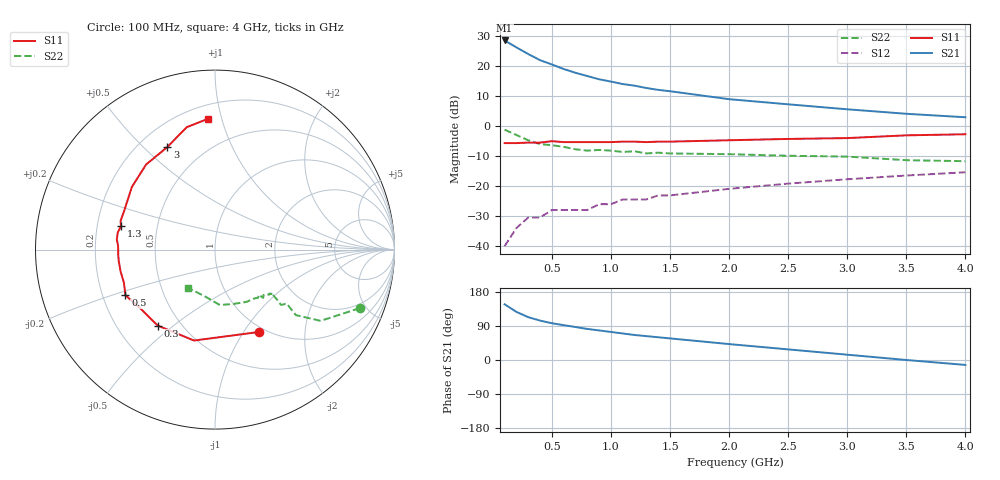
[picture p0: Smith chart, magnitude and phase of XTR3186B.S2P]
! HXTR-3186
! Typical S-Parameters Vce = 10 V, Ic = 15 mA
# ghz s ma r 50
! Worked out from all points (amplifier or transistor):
!   20 points, 100 MHz to 4 GHz, reference 50 ohm
!   highest |S21| = 28.5 dB at 100 MHz (marker M1)
!   |S21| within 3 dB of that: start of sweep to 231.3 MHz
!   unconditionally stable (mu >= 1): 773.1 MHz to 835.6 MHz; 974.3 MHz to 1.031 GHz; 1.205 GHz to 3.226 GHz
!   at 400 MHz: K = 0.67, MSG = 26.2 dB, |S12| = -30.5 dB
!   at 1.1 GHz: K = 0.95, MSG = 19.2 dB, |S12| = -24.4 dB
!   at 4 GHz: K = 0.91, MSG = 9.2 dB, |S12| = -15.4 dB
!   S11 on the Smith chart (normalised r, x): 100 MHz: 0.93, -1.17; 300 MHz: 0.37, -0.44; 500 MHz: 0.30, -0.22; 1.3 GHz: 0.30, +0.11; 3 GHz: 0.31, +0.59; 4 GHz: 0.29, +0.91
0.1  0.52 -62.0  26.6 147.0  0.01 66.0  0.87 -22.0
0.2  0.52 -103.0  20.4 127.0  0.02 55.0  0.71 -34.0
0.3  0.53 -127.0  15.8 113.0  0.03 49.0  0.58 -39.0
0.4  0.53 -142.0  12.5 104.0  0.03 48.0  0.5 -37.0
0.5  0.56 -153.0  10.6 97.0  0.04 47.0  0.48 -40.0
0.6  0.54 -160.0  8.9 92.0  0.04 49.0  0.45 -39.0
0.7  0.54 -167.0  7.7 87.0  0.04 49.0  0.41 -38.0
0.8  0.54 -173.0  6.8 82.0  0.04 50.0  0.39 -39.0
0.9  0.54 -177.0  6 78.0  0.05 51.0  0.4 -38.0
1  0.54 178.0  5.5 74.0  0.05 52.0  0.39 -40.0
1.1  0.55 174.0  5 70.0  0.06 52.0  0.37 -43.0
1.2  0.55 170.0  4.7 66.0  0.06 52.0  0.38 -45.0
1.3  0.54 166.0  4.3 63.0  0.06 52.0  0.35 -46.0
1.4  0.55 163.0  4 60.0  0.07 52.0  0.36 -48.0
1.5  0.55 157.0  3.8 57.0  0.07 52.0  0.35 -51.0
2  0.58 143.0  2.8 42.0  0.09 50.0  0.34 -59.0
2.5  0.61 129.0  2.3 28.0  0.11 46.0  0.32 -71.0
3  0.63 115.0  1.9 14.0  0.13 41.0  0.31 -85.0
3.5  0.7 103.0  1.6 0.0  0.15 35.0  0.27 -100.0
4  0.73 93.0  1.4 -13.0  0.17 29.0  0.26 -125.0
